|   This file is an IBIS representation of the   |
|   Integrated Device Technology Inc   |
|   IDT8T49N286   |
|   FEMTOCLOCK NG OCTAL UNIVERSAL FREQUENCY TRANSLATOR   |
[IBIS Ver]   4.1
[File name]   8t49n286i.ibs
[File Rev]   1.0
[Date]   04 Dec 2014
[Source]   Originated at Integrated Device Technology, Inc.
[Disclaimer]
IDT hereby grants the user of this IBIS model a non-exclusive,
nontransferable license to use this IBIS model under the following terms.
Before using this IBIS model, the user should read this license.
If the user does not accept these terms,  the IBIS model should be
returned to IDT within 30 days.
   The user is granted this license only to use the IBIS model and
is not granted rights to sell, load, rent, lease or license the IBIS
model in whole or in part, or in modified form to anyone other than
user. User may modify the IBIS model to suit its specific
applications but rights to derivative works and such modifications
shall belong to IDT.
   This IBIS model is provided on an "AS IS" basis and IDT makes
absolutely no warranty with respect to the information contained
herein. IDT DISCLAIMS AND CUSTOMER WAIVES ALL WARRANTIES, EXPRESS
OR IMPLIED, INCLUDING WARRANTIES OF MERCHANTABILITY OR FITNESS FOR
A PARTICULAR PURPOSE. The entire risk as to quality and performance
is with the Customer. ACCORDINGLY, IN NO EVENT SHALL THE COMPANY BE
LIABLE FOR ANY DAMAGES, WHETHER IN CONTRACT OR TORT,INCLUDING ANY
LOST PROFITS OR OTHER INCIDENTAL, CONSEQUENTIAL, EXEMPLARY, OR
PUNITIVE DAMAGES ARISING OUT OF THE USE OR APPLICATION OF THE IBIS
model provided in this package. Further, IDT reserves the right to
make changes without notice to any product herein to improve
reliability, function, or design. IDT does not convey any license
under patent rights or any other intellectual property rights,
including those of third parties.
   IDT is not obligated to provide maintenance or support
for the licensed IBIS model.
[Copyright] Copyright 2014 by Integrated Device Technology, Inc.
[Component]   IDT8T49N286NLI
[Manufacturer] Integrated Device Technology, Inc.
[Package]
|LD QFN 72
|lead + wire
|   Typ   Min   Max
R_pkg   7.8601440E-02   3.3809435E-02   1.3219826E-01
L_pkg   2.3894137E-09   1.4510419E-09   3.7197948E-09
C_pkg   6.1248861E-13   5.1617034E-13   1.0239547E-12
[Pin] signal_name model_name   R_pin   L_pin   C_pin
1  VCCA   POWER   1.0433593E-01   2.9865323E-09   5.7909691E-13
2  OSCI   CAK_INESD01   9.7880543E-02   2.8166436E-09   5.6666836E-13
3  OSCO   NC   5.1811148E-02   1.8446542E-09   7.0153751E-13
4  NC   NC   4.9278689E-02   1.7780066E-09   6.8203455E-13
5  S_A0/nCS   CAK_INESD02_PD   8.6539992E-02   2.5181904E-09   5.4483440E-13
6  VEE   GND   8.4441065E-02   2.4629522E-09   5.4079334E-13
7  CLK0   CAK_INESD02_PD   8.4441065E-02   2.4629522E-09   5.4079334E-13
8  nCLKO   CAK_INESD02_PMID   4.8919175E-02   1.7685452E-09   6.7926586E-13
9  CLK1   CAK_INESD02_PD   4.9434655E-02   1.7821112E-09   6.8323567E-13
10 nCLK1   CAK_INESD02_PMID   5.0386309E-02   1.8071563E-09   6.9056455E-13
11 CLK2   CAK_INESD02_PD   5.0423318E-02   1.8081302E-09   6.9084956E-13
12 nCLK2   CAK_INESD02_PMID   5.1361755E-02   1.8328274E-09   6.9807665E-13
13 CLK3   CAK_INESD02_PD   9.0616246E-02   2.6254666E-09   5.5268241E-13
14 nCLK3   CAK_INESD02_PMID   5.4338319E-02   1.9111627E-09   7.2099976E-13
15 VCC   POWER   5.7534293E-02   1.9952722E-09   7.4561258E-13
16 SDATA/SDO   CAK_IOCMOS35OHM0   1.0684196E-01   3.0524842E-09   5.8392176E-13
17 SCLK/SCLK   CAK_IOCMOS35OHM0   6.3794065E-02   2.1600128E-09   7.9382033E-13
18 S_A1/SDI   CAK_INESD01_PD   6.8504756E-02   2.2839856E-09   8.3009828E-13
19 VCCA   POWER   1.3219826E-01   3.7197948E-09   6.3274024E-13
20 VCCA   POWER   1.1609415E-01   3.2959774E-09   6.0173501E-13
21 VCCA   POWER   7.5182199E-02   2.4597182E-09   8.8152259E-13
22 VCCA   POWER   6.9112757E-02   2.2999866E-09   8.3478062E-13
23 CAP1   NC   1.1068558E-01   3.1536382E-09   5.9132189E-13
24 CAP1_REF   NC   1.0047644E-01   2.8849608E-09   5.7166624E-13
25 VCCA   POWER   9.3143418E-02   2.6919750E-09   5.5754797E-13
26 GPI01   CAK_IOCMOS25OHM0   8.5715225E-02   2.4964847E-09   5.4324648E-13
27 VCCO3   POWER   4.6492456E-02   1.7046804E-09   6.6057722E-13
28 Q3   CAK_OCELL_MULTOUT   4.4242850E-02   1.6454767E-09   6.4325256E-13
29 nQ3   CAK_OCELL_MULTOUT   7.3021210E-02   2.1624120E-09   5.1880670E-13
30 VEE   GND   7.3058219E-02   2.1633860E-09   5.1887795E-13
31 GPIO0   CAK_IOCMOS25OHM0   7.3338428E-02   2.1707603E-09   5.1941744E-13
32 nI2C_SPI   CAK_INESD01_PD_5   7.3808968E-02   2.1831437E-09   5.2032337E-13
33 VCCO2   POWER   8.4351186E-02   2.4605869E-09   5.4062029E-13
34 Q2   CAK_OCELL_MULTOUT   9.5194762E-02   2.7459609E-09   5.6149742E-13
35 nQ2   CAK_OCELL_MULTOUT   1.0813726E-01   3.0865732E-09   5.8641562E-13
36 VEE   GND   6.5747601E-02   2.2114246E-09   8.0886489E-13
37 GPIO3   CAK_IOCMOS25OHM0   4.9113451E-02   1.8538029E-09   1.0239547E-12
38 nQ7   CAK_OCELL_MULTOUT   9.7737794E-02   2.8128868E-09   5.6639352E-13
39 Q7   CAK_OCELL_MULTOUT   9.2530129E-02   2.6758349E-09   5.5636721E-13
40 VCCO7   POWER   9.2128319E-02   2.6652603E-09   5.5559360E-13
41 GPIO7   CAK_IOCMOS25OHM0   9.3656254E-02   2.7054715E-09   5.5853533E-13
42 nQ6   CAK_OCELL_MULTOUT   8.7877595E-02   2.5533926E-09   5.4740969E-13
43 Q6   CAK_OCELL_MULTOUT   4.9646134E-02   1.7876768E-09   6.8486431E-13
44 VCCO6   POWER   8.2659356E-02   2.4160624E-09   5.3736301E-13
45 GPIO6   CAK_IOCMOS25OHM0   8.3494697E-02   2.4380463E-09   5.3897130E-13
46 nQ5   CAK_OCELL_MULTOUT   3.7649538E-02   1.5521032E-09   8.2531156E-13
47 Q5   CAK_OCELL_MULTOUT   8.4081551E-02   2.4534908E-09   5.4010117E-13
48 VCCO5   POWER   8.3891220E-02   2.4484818E-09   5.3973472E-13
49 GPIO5   CAK_IOCMOS25OHM0   8.3351949E-02   2.4342896E-09   5.3869646E-13
50 nQ4   CAK_OCELL_MULTOUT   8.5186528E-02   2.4825708E-09   5.4222858E-13
51 Q4   CAK_OCELL_MULTOUT   9.1160804E-02   2.6397979E-09   5.5373085E-13
52 VCCO4   POWER   9.8874493E-02   2.8428017E-09   5.6858201E-13
53 GPIO4   CAK_IOCMOS25OHM0   1.0953831E-01   3.1234451E-09   5.8911305E-13
54 GPIO2   CAK_IOCMOS25OHM0   1.2195212E-01   3.4501434E-09   6.1301334E-13
55 VEE   GND   1.2167719E-01   3.4429082E-09   6.1248403E-13
56 nQ1   CAK_OCELL_MULTOUT   8.8147231E-02   2.5604887E-09   5.4792882E-13
57 Q1   CAK_OCELL_MULTOUT   7.9159382E-02   2.3239524E-09   5.3062452E-13
58 VCCO1   POWER   7.4469839E-02   2.2005361E-09   5.2159574E-13
59 nWP   CAK_INESD01_PU_5   7.7462265E-02   2.2792887E-09   5.2735706E-13
60 nRST   CAK_INESD01_PU_5   4.4171476E-02   1.6435984E-09   6.4270289E-13
61 VEE   GND   3.3809435E-02   1.4510419E-09   7.5877144E-13
62 nQ0   CAK_OCELL_MULTOUT   7.5040832E-02   2.2155631E-09   5.2269508E-13
63 Q0   CAK_OCELL_MULTOUT   7.4718327E-02   2.2070756E-09   5.2207416E-13
64 VCCO0   POWER   7.1651884E-02   2.1263750E-09   5.1617034E-13
65 nINT   OUTPUT_OD01   4.4782121E-02   1.6596689E-09   6.4740559E-13
66 VCCA   POWER   4.5897672E-02   1.6890272E-09   6.5599667E-13
67 CAP0_REF   NC   8.0169193E-02   2.3505279E-09   5.3256871E-13
68 CAP0   NC   7.4554431E-02   2.2027623E-09   5.2175861E-13
69 PLL_BYP   CAK_INESD01_PD_5   8.1015108E-02   2.3727901E-09   5.3419735E-13
70 VCCA   POWER   8.9516556E-02   2.5965257E-09   5.5056518E-13
71 VCCA   POWER   9.8779328E-02   2.8402972E-09   5.6839879E-13
72 VCCA   POWER   1.0886687E-01   3.1057744E-09   5.8782032E-13
[Diff Pin]   inv_pin vdiff   tdelay_typ   tdelay_min   tdelay_max
| Inputs
7   8   150mV   NA   NA   NA
9   10   150mV   NA   NA   NA
11   12   150mV   NA   NA   Na
13   14   150mV   NA   NA   NA
|Outputs
28   29   NA   0   0   0
34   35   NA   0   0   0
39   38   NA   0   0   0
43   42   NA   0   0   0
47   46   NA   0   0   0
51   50   NA   0   0   0
57   56   NA   0   0   0
63   62   NA   0   0   0
[Model Selector] CAK_INESD01
CAK_INESD01_2v5   Buffer selection for 2v5
CAK_INESD01_3v3   Buffer selection for 3v3
[Model Selector] CAK_INESD02_PD
CAK_INESD02_PD_2v5  Buffer selection for 2v5
CAK_INESD02_PD_3v3  Buffer selection for 3v3
[Model Selector] CAK_INESD02_PMID
CAK_INESD02_PMID_2v5  Buffer selection for 2v5
CAK_INESD02_PMID_3v3  Buffer selection for 3v3
[Model Selector] CAK_IOCMOS35OHM0
CAK_IOCMOS35OHM0_2v5  Buffer selection for 2v5
CAK_IOCMOS35OHM0_3v3  Buffer selection for 3v3
[Model Selector] CAK_IOCMOS25OHM0
CAK_IOCMOS25OHM0_2v5  Buffer selection for 2v5
CAK_IOCMOS25OHM0_3v3  Buffer selection for 3v3
[Model Selector] CAK_OCELL_MULTOUT
CAK_OCELL_LVPECL_2v5  Buffer selection for LVPECL 2.5V
CAK_OCELL_LVPECL_3v3  Buffer selection for LVPECL 3.3V
CAK_OCELL_LVDS_2v5   Buffer selection for LVDS 2.5V
CAK_OCELL_LVDS_3v3   Buffer selection for LVDS 3.3V
CAK_OCELL_CMOS_1v8   Buffer selection for CMOS 1.8V
CAK_OCELL_CMOS_2v5   Buffer selection for CMOS 2.5V
CAK_OCELL_CMOS_3v3   Buffer selection for CMOS 3.3V
CAK_OCELL_HCSL_2v5   Buffer selection for HCSL 2.5V
CAK_OCELL_HCSL_3v3   Buffer selection for HCSL 3.3V
[Model Selector] CAK_INESD01_PU_5
CAK_INESD01_PU_5_2v5  Buffer selection for 2v5
CAK_INESD01_PU_5_3v3  Buffer selection for 3v3
[Model Selector] OUTPUT_OD01
OUTPUT_OD01_2v5  Buffer selection for 2v5
OUTPUT_OD01_3v3  Buffer selection for 3v3
[Model Selector] CAK_INESD01_PD_5
CAK_INESD01_PD_5_2v5  Buffer selection for 2v5
CAK_INESD01_PD_5_3v3  Buffer selection for 3v3
[Model Selector] CAK_INESD01_PD
CAK_INESD01_PD_2v5  Buffer selection for 2v5
CAK_INESD01_PD_3v3  Buffer selection for 3v3
| Models and submodels in the file (27): CAK_INESD01_3v3 (Input), CAK_INESD01_2v5 (Input), CAK_OCELL_CMOS_1v8 (Output), CAK_INESD02_PD_2v5 (Input), CAK_INESD02_PMID_2v5 (Input), CAK_IOCMOS35OHM0_2v5 (I/O), CAK_IOCMOS25OHM0_2v5 (I/O), CAK_OCELL_LVPECL_2v5 (Output_ECL), CAK_OCELL_CMOS_2v5 (Output), CAK_OCELL_LVDS_2v5 (Output), CAK_INESD01_PU_5_2v5 (Input), OUTPUT_OD01_2v5 (Open_drain), CAK_INESD01_PD_5_2v5 (Input), CAK_INESD02_PD_3v3 (Input), CAK_INESD02_PMID_3v3 (Input), CAK_IOCMOS35OHM0_3v3 (Output), CAK_IOCMOS25OHM0_3v3 (I/O), CAK_OCELL_LVPECL_3v3 (Output_ECL), CAK_OCELL_CMOS_3v3 (Output), CAK_OCELL_LVDS_3v3 (Output), CAK_INESD01_PU_5_3v3 (Input), OUTPUT_OD01_3v3 (Open_drain), CAK_INESD01_PD_5_3v3 (Input), CAK_INESD01_PD_3v3 (Input), CAK_INESD01_PD_2v5 (Input), CAK_OCELL_HCSL_3v3 (Open_source), CAK_OCELL_HCSL_2v5 (Open_source)
